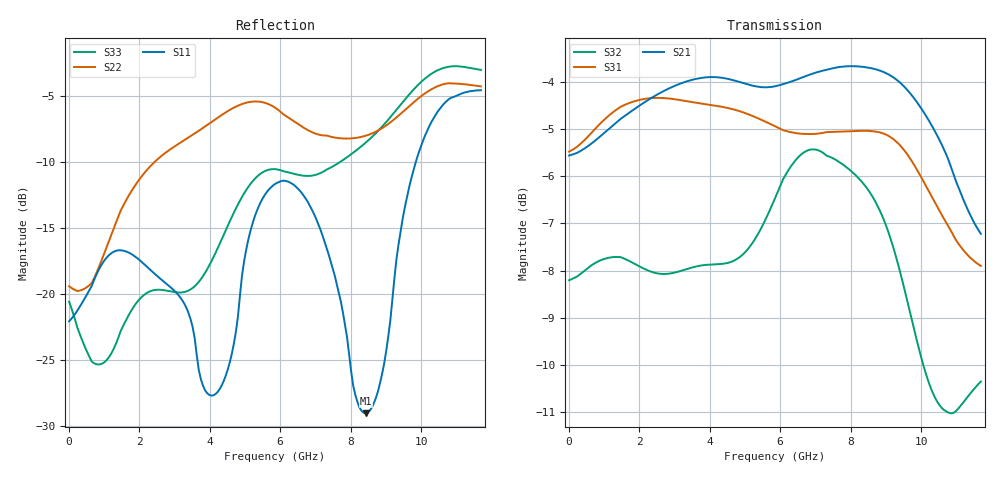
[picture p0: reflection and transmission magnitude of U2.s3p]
!Keysight Technologies,N5247A,US50470148,Z.10.63.25
!Date: Wednesday, May 22, 2019 07:34:10
!Correction: S11(Full 3 Port(1,2,3))
!S12(Full 3 Port(1,2,3))
!S13(Full 3 Port(1,2,3))
!S21(Full 3 Port(1,2,3))
!S22(Full 3 Port(1,2,3))
!S23(Full 3 Port(1,2,3))
!S31(Full 3 Port(1,2,3))
!S32(Full 3 Port(1,2,3))
!S33(Full 3 Port(1,2,3))
!S3P File: Measurements: <S11,S12,S13>,
!<S21,S22,S23>,
!<S31,S32,S33>:
# Hz S  dB  R 50
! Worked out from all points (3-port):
!   201 points, 10 MHz to 11.7 GHz, reference 50 ohm
!   strongest paths, dB at 10 MHz, 2.933 GHz, 5.855 GHz, 8.777 GHz, 11.7 GHz:
!     S21: -5.6, -4.1, -4.1, -3.8, -7.2
!     S31: -5.5, -4.4, -4.9, -5.1, -7.9
!     S32: -8.2, -8.1, -6.5, -6.6, -10.3
!   lowest |S11| = -29.1 dB at 8.427 GHz (marker M1), VSWR 1.07, Z = 50.8 - j3.45 ohm
!   |S11| at or under -10 dB: start of sweep to 9.855 GHz
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1e7  -22.09 27.7  -5.55 176.2  -5.49 -1.7
     -5.57 176.2  -19.44 136.0  -8.26 2.6
     -5.48 -1.9  -8.20 2.3  -20.60 146.1
8.8675e8  -18.00 -25.8  -5.15 151.5  -4.89 -20.7
          -5.16 151.4  -17.77 77.8  -7.80 -6.6
          -4.89 -20.7  -7.79 -6.6  -25.36 91.0
2.9325e9  -19.61 -131.5  -4.09 79.6  -4.35 -81.6
          -4.12 79.5  -8.97 -8.1  -8.07 -19.9
          -4.37 -81.6  -8.05 -19.9  -19.85 -4.7
4.2184e9  -27.47 76.1  -3.88 35.0  -4.50 -121.8
          -3.91 34.9  -6.68 -49.9  -7.88 -28.3
          -4.52 -121.7  -7.86 -28.2  -16.61 -44.8
5.1536e9  -15.28 -41.8  -4.05 4.4  -4.70 -152.3
          -4.08 4.4  -5.46 -77.9  -7.49 -33.7
          -4.71 -152.3  -7.48 -33.7  -11.70 -63.9
5.855e9  -11.69 -55.7  -4.08 -17.4  -4.94 -176.0
         -4.10 -17.4  -5.90 -91.3  -6.48 -38.7
         -4.95 -175.9  -6.47 -38.7  -10.56 -69.9
7.1409e9  -15.11 -82.0  -3.77 -58.5  -5.09 139.3
          -3.78 -58.6  -7.97 -106.0  -5.48 -62.3
          -5.10 139.4  -5.47 -62.2  -10.86 -70.9
8.4268e9  -29.07 -74.4  -3.68 -102.5  -5.03 88.4
          -3.70 -102.5  -8.03 -108.4  -6.23 -86.8
          -5.04 88.4  -6.22 -86.7  -8.56 -77.8
1.000495e10  -8.78 -37.1  -4.55 -162.6  -6.02 20.0
             -4.57 -162.7  -5.03 -115.7  -9.84 -106.7
             -6.02 19.9  -9.83 -106.6  -3.95 -106.5
1.17e10  -4.58 -67.0  -7.20 140.1  -7.90 -30.9
         -7.22 140.0  -4.29 -149.7  -10.36 -110.2
         -7.90 -30.9  -10.35 -110.0  -3.04 -135.7
